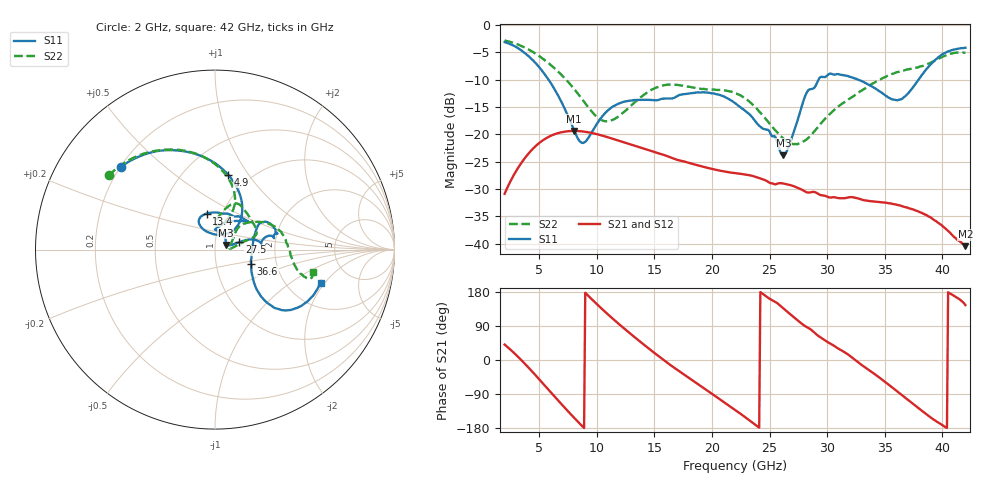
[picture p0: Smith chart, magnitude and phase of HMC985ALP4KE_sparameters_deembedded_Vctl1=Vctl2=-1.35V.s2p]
!s2p File: Measurements: S11, S21, S12, S22
# GHz S dB R 50.0
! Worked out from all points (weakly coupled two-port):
!   401 points, 2 GHz to 42 GHz, reference 50 ohm
!   highest |S21| = -19.37 dB at 8 GHz (marker M1); lowest = -40.4 dB at 42 GHz (marker M2)
!   lowest |S11| = -23.8 dB at 26.2 GHz (marker M3), VSWR 1.14, Z = 56.2 + j2.9 ohm
!   |S11| at or under -10 dB: 5.813 GHz to 29.25 GHz (23.43 GHz wide, 134 % of centre); 32.69 GHz to 37.93 GHz (5.239 GHz wide, 14.8 % of centre)
!   |S22| runs from -21.8 to -2.8 dB; largest |S21 - S12| = 0.00017
!   S11 on the Smith chart (normalised r, x): 2 GHz: 0.20, +0.36; 4.9 GHz: 0.79, +0.81; 13.4 GHz: 0.84, +0.35; 27.5 GHz: 1.31, +0.11; 36.6 GHz: 1.48, -0.25; 42 GHz: 3.06, -1.84
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2  -3.12 138.5  -30.86 40.8  -30.86 40.7  -2.83 145.1
3.4  -4.58 110.8  -25.38 1.3  -25.39 1.3  -3.78 122.1
4.9  -7.46 80.1  -21.75 -47.4  -21.76 -47.4  -5.53 98.5
6.2  -11.27 56.2  -20.08 -91.7  -20.09 -91.7  -7.66 80.7
8  -19.13 53.3  -19.37 -151.4  -19.38 -151.4  -11.59 66.0
8.7  -21.54 79.4  -19.45 -173.4  -19.45 -173.4  -13.48 65.7
10.8  -15.95 121.8  -20.42 125.0  -20.42 125.0  -17.60 84.0
13.4  -13.71 102.9  -22.13 57.4  -22.14 57.4  -13.94 81.3
15.4  -13.67 76.3  -23.49 9.6  -23.49 9.6  -11.26 68.7
18.9  -12.34 40.7  -25.73 -66.2  -25.74 -66.2  -11.61 42.2
22  -14.27 55.5  -27.07 -131.4  -27.09 -131.5  -12.43 19.3
24.5  -19.01 89.7  -28.27 172.4  -28.28 172.4  -16.74 13.5
26.2  -23.80 23.4  -28.98 136.1  -28.99 136.1  -20.77 4.3
27.5  -16.95 17.0  -29.82 102.9  -29.82 102.8  -21.70 7.3
28.2  -12.48 12.5  -30.57 87.3  -30.57 87.4  -20.94 16.6
28.7  -11.69 8.0  -30.53 77.6  -30.54 77.7  -19.89 23.6
31.1  -9.07 19.6  -31.67 27.9  -31.67 27.9  -14.69 43.6
33.3  -10.57 30.4  -32.06 -19.4  -32.08 -19.4  -11.59 35.7
35.4  -13.34 9.8  -32.60 -66.7  -32.59 -66.7  -9.18 22.8
36.6  -13.31 -21.5  -33.18 -95.2  -33.16 -95.2  -8.34 13.9
39.6  -6.01 -42.3  -36.12 -164.2  -36.08 -164.1  -6.25 -15.0
42  -4.16 -17.4  -40.44 144.9  -40.47 144.9  -5.07 -12.8
